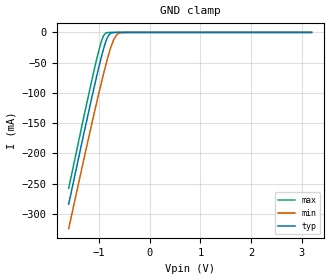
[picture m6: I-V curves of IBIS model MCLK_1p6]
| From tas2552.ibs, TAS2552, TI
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|   Model
[Model]   MCLK_1p6
Model_type   Input
Vinl = 0.48
Vinh = 1.12
|   typ   min   max
C_comp   1.014pF   0.983pF   1.069pF
[Voltage Range]   1.6   1.5   1.7
[Temperature Range]   27   125   -40
[Power Clamp Reference]   1.6   1.5   1.7
[GND Clamp Reference]   -0   -0   -0
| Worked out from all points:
|   GND clamp passes 1 mA (typ) near -0.76 V on its own axis
[GND Clamp]
|   Voltage   I(typ)   I(min)   I(max)
-1.6V     -283.7mA   -324.1mA   -257.5mA
-1.125V   -100.7mA   -143.9mA   -72.23mA
-961.6mV  -43.02mA   -85.41mA   -16.99mA
-899.2mV  -23.81mA   -64.22mA   -3.871mA
-856mV    -12.78mA   -50.22mA   -803.8uA
-812.8mV  -5.049mA   -37.03mA   -230.6uA
-774.4mV  -1.627mA   -26.31mA   -136.7uA
-707.2mV  -174.9uA   -11.15mA   -80.52uA
-640mV    -29.18uA   -2.895mA   -42.78uA
-572.8mV  -7.176uA   -500.3uA   -16.69uA
-400mV    -97.63nA   -3.636uA   -222.8nA
3.195V    0A         0A         0A
[POWER Clamp]
|   Voltage   I(typ)   I(min)   I(max)
-1.6V     0A         0A         0A
-1.59V    0A         0A         0A
-1.586V   0A         0A         0A
3.195V    0A         0A         0A
